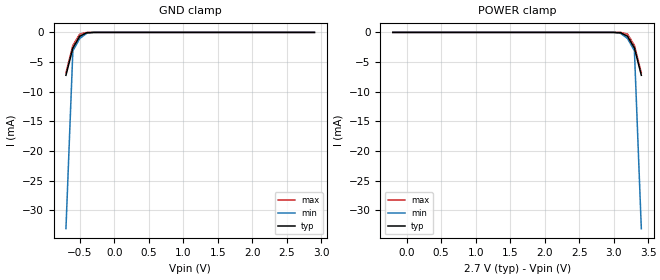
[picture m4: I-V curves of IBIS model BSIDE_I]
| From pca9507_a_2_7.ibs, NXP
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[Model]   BSIDE_I
Model_type Input
Vinh=1.89
Vinl=0.81
C_comp   4.8p   4.6p   5p
[Temperature Range] 27   85   -40
[Voltage Range]   2.7   2.5   2.9
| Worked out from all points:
|   GND clamp passes 1 mA (typ) near -0.52 V on its own axis
[GND Clamp]
-700mV    -7.237mA   -33.11mA   -6.803mA
-600mV    -2.643mA   -3.103mA   -2.2mA
-500mV    -659.2uA   -1.029mA   -279.4uA
-400mV    -54.1uA    -160uA     -7.517uA
-300mV    -1.452uA   -7.642uA   -78.66nA
2.9V      185.3pA    333.6pA    173.2pA
[POWER Clamp]
-200mV    185.3pA    333.6pA    173.2pA
3V        -1.452uA   -7.642uA   -78.66nA
3.1V      -54.1uA    -160uA     -7.517uA
3.2V      -659.2uA   -1.029mA   -279.4uA
3.3V      -2.643mA   -3.103mA   -2.2mA
3.4V      -7.237mA   -33.11mA   -6.803mA
